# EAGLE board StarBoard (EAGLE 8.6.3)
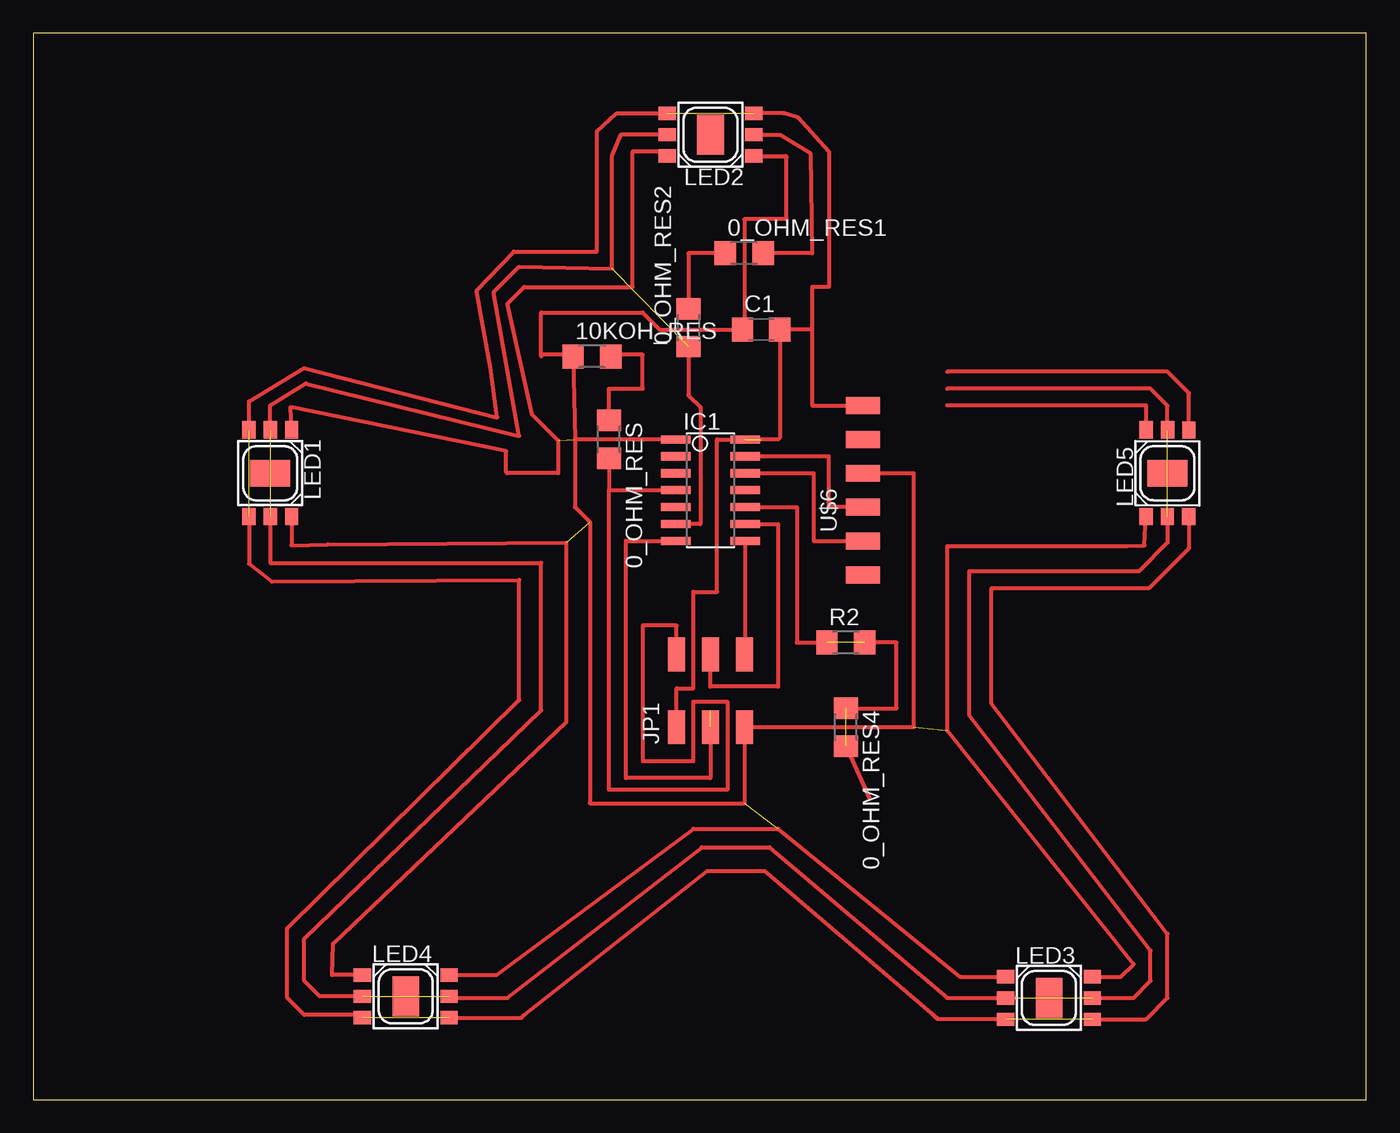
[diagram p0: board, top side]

Size 100 x 80 mm. Coordinates in mm from the lower left corner, seen from the top.
Outline: 0,0 100,0 100,80 0,80 0,0
Copper layers (1*16): Top 0.035mm / dielectric 1.5mm / Bottom 0.035mm
Design rules "default": minimum track width 6mil, minimum drill 0.35mm, track to track 6mil, track to pad 6mil, pad to pad 6mil, via to via 6mil, smd to smd 6mil, copper to edge 40mil, drill to drill 6mil, minimum pad ring 10mil, minimum via ring 8mil, stop-mask expansion 4mil, vias tented up to drill 0mil, thermal gap 10mil

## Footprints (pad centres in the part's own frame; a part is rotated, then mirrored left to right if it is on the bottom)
R1206 = smd 1.6 x 1.803: 1 -1.422,0; 2 1.422,0
C1206 = smd 1.6 x 1.8: 1 -1.4,0; 2 1.4,0
SOIC14 = smd 0.61 x 2.21: 1 -3.81,-2.603; 2 -2.54,-2.603; 3 -1.27,-2.603; 4 0,-2.603; 5 1.27,-2.603; 6 2.54,-2.603; 7 3.81,-2.603; 8 3.81,2.603; 9 2.54,2.603; 10 1.27,2.603; 11 0,2.603; 12 -1.27,2.603; 13 -2.54,2.603; 14 -3.81,2.603
2X03SMD = smd 2.54 x 1.27: 1 -2.54,2.54; 2 2.92,2.54; 3 -2.54,0; 4 2.92,0; 5 -2.54,-2.54; 6 2.92,-2.54
LP2C63-ST-RGB-SR0 = smd 1.3 x 1: 1 -3.25,1.6; 2 -3.25,0; 3 -3.25,-1.6; 4 3.25,-1.6; 5 3.25,0; 6 3.25,1.6 | smd 2 x 3: TH 0,0
1X06SMD = smd 2.54 x 1.27: 1 0,6.35; 2 0,3.81; 3 0,1.27; 4 0,-1.27; 5 0,-3.81; 6 0,-6.35

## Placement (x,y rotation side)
0_OHM_RES  [R1206]  43.18,49.53 270 top
0_OHM_RES1  [R1206]  53.34,63.5 0 top
0_OHM_RES2  [R1206]  49.15,57.91 90 top
0_OHM_RES4  [R1206]  60.96,27.94 270 top
10KOH_RES  [R1206]  41.91,55.75 0 top
C1  CAP-US1206  [C1206]  54.61,57.78 0 top
IC1  ATTINY44-SSU  [SOIC14]  50.8,45.72 270 top
JP1  [2X03SMD]  50.8,30.48 90 top
LED1  LP2C63-ST-RGB-SR0  [LP2C63-ST-RGB-SR0]  17.78,46.99 270 top
LED2  LP2C63-ST-RGB-SR0  [LP2C63-ST-RGB-SR0]  50.8,72.39 180 top
LED3  LP2C63-ST-RGB-SR0  [LP2C63-ST-RGB-SR0]  76.2,7.62 0 top
LED4  LP2C63-ST-RGB-SR0  [LP2C63-ST-RGB-SR0]  27.94,7.75 0 top
LED5  LP2C63-ST-RGB-SR0  [LP2C63-ST-RGB-SR0]  85.09,46.99 89.9 top
R2  [R1206]  60.96,34.29 0 top
U$6  FTDI-SMD-HEADER  [1X06SMD]  62.23,45.72 0 top

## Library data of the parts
0_OHM_RES 0_OHM_RES1 0_OHM_RES2 0_OHM_RES4 10KOH_RES C1 IC1 JP1 R2 U$6 = fab
LED1-LED5 = led

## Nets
GND: C1.2 IC1.14 JP1.1 LED1.3 LED1.4 LED2.3 LED2.4 LED3.3 LED3.4 LED4.3 LED4.4 LED5.3 U$6.1
N$1: IC1.8 JP1.6
N$5: 0_OHM_RES.1 10KOH_RES.2
N$7: IC1.12 U$6.5
N$8: IC1.13 U$6.4
N$9: IC1.7 JP1.3
N$10: IC1.9 JP1.4
N$16: LED5.6
N$19: 0_OHM_RES1.2 LED2.2
N$24: 0_OHM_RES1.1 0_OHM_RES2.2
N$26: LED5.4
PA3: 0_OHM_RES4.1 0_OHM_RES4.2 IC1.10 R2.1 R2.2
PA7: 0_OHM_RES2.1 IC1.6 LED1.2 LED1.5 LED2.5 LED3.2 LED3.5 LED4.2 LED4.5 LED5.2 LED5.5
REST: 0_OHM_RES.2 IC1.4 JP1.2
VCC: 10KOH_RES.1 C1.1 IC1.1 JP1.5 LED1.1 LED1.6 LED2.1 LED2.6 LED3.1 LED3.6 LED4.1 LED4.6 LED5.1 U$6.3

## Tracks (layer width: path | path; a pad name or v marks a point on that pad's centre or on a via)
GND  (5 unrouted)
  Top 0.305: IC1.14 51.31,49.53 51.31,38.1 49.53,38.1 49.53,30.86 48.26,30.86 JP1.1 | 54.61,49.53 55.88,49.53 56.01,49.66 C1.2 58.42,57.78 | 58.42,57.78 58.42,60.96 59.69,60.96 59.69,71.12 57.4,73.66 56.31,73.99 LED2.3 | 58.42,57.78 58.42,52.07 U$6.1 | LED1.3 16.18,52.38 20.32,54.86 34.8,51.18 34.29,54.86 33.27,60.71 36.07,63.63 42.29,63.63 42.29,72.64 43.76,73.99 LED2.4 | LED4.3 24.49,6.35 20.32,6.35 19.05,7.62 19.05,12.83 36.45,29.97 36.45,38.99 17.91,38.86 16.18,40.21 LED1.4 | LED4.4 36.63,6.15 36.83,6.35 50.55,17.14 54.86,17.14 67.4,6.45 | 67.82,6.1 67.4,6.45 | LED3.3 67.83,6.02 67.4,6.45 | LED3.4 83.49,6.02 85.09,7.62 85.09,12.45 71.88,29.72 71.88,38.35 83.69,38.35 86.68,41.34 LED5.3 86.36,43.41
N$1
  Top 0.305: IC1.8 53.4,33.4 JP1.6
N$5
  Top 0.305: 0_OHM_RES.1 43.18,53.34 45.72,53.34 45.72,55.88 43.46,55.88 10KOH_RES.2
N$7
  Top 0.305: IC1.12 58.55,46.99 58.55,41.91 U$6.5
N$8
  Top 0.305: U$6.4 59.69,44.45 59.69,48.26 IC1.13
N$9  (1 unrouted)
  Top 0.305: JP1.3 50.8,24.13 44.45,24.13 44.45,41.91 IC1.7
N$10
  Top 0.305: IC1.9 55.88,43.18 55.88,30.99 50.8,30.99 JP1.4
N$16
  Top 0.305: LED5.6 83.5,52.07 68.58,52.07
N$19
  Top 0.305: LED2.2 56.01,72.39 58.29,70.99 58.42,63.5 0_OHM_RES1.2
N$24
  Top 0.305: 0_OHM_RES1.1 49.15,63.5 0_OHM_RES2.2
N$26
  Top 0.305: LED5.4 86.7,53 85.09,54.61 68.58,54.61
PA3  (2 unrouted)
  Top 0.305: IC1.10 57.28,44.45 57.28,34.29 R2.1 | R2.2 64.77,34.29 64.77,29.36 0_OHM_RES4.1 | 0_OHM_RES4.2 62.74,22.61
PA7  (5 unrouted)
  Top 0.305: IC1.6 50.04,43.18 50.04,51.94 49.15,52.83 0_OHM_RES2.1 | LED2.5 44.07,72.39 43.43,70.87 43.43,62.36 36.45,62.48 34.54,60.58 36.45,49.78 20.45,53.72 17.78,52.07 LED1.2 | LED4.2 21.46,7.75 20.32,8.89 20.32,12.06 38.1,29.21 38.1,40.26 17.78,40.26 LED1.5 | LED4.5 31.32,7.62 35.56,7.62 50.16,18.92 55.24,18.92 68.58,7.62 LED3.2 73.66,7.62 | LED3.5 82.55,7.62 83.82,8.89 83.82,11.18 70.23,28.83 70.23,39.62 82.93,39.62 85.08,41.78 LED5.2 | LED5.5 85.1,52.06 83.82,53.34 68.58,53.34
REST
  Top 0.305: 0_OHM_RES.2 43.18,45.72 | 43.18,45.72 IC1.4 | JP1.2 48.26,35.56 45.72,35.56 45.72,25.4 49.53,25.4 49.53,29.84 52.07,29.84 52.07,23.24 43.18,23.24 43.18,45.72
VCC  (4 unrouted)
  Top 0.305: U$6.3 66.04,46.99 66.04,27.94 JP1.5 53.34,22.23 41.76,22.23 41.76,43.33 40.64,44.45 40.64,49.53 | 38.1,55.75 38.1,55.88 | 38.1,55.88 38.1,59.05 45.72,59.05 46.99,57.78 C1.1 53.34,57.78 53.34,66.04 56.52,66.04 56.52,70.74 56.46,70.79 LED2.1 | 40.64,49.53 10KOH_RES.1 40.36,55.88 38.1,55.88 | IC1.1 40.64,49.53 | LED2.6 47.22,71.12 44.96,71.12 44.96,60.96 36.83,60.96 35.56,59.69 37.4,51.41 39.37,49.44 39.37,46.99 35.56,46.99 35.48,47.07 35.48,48.65 19.3,51.94 LED1.1 | LED4.1 22.4,9.35 22.48,11.68 40.01,28.32 40.01,41.78 22.1,41.66 19.38,41.58 LED1.6 | LED4.6 34.75,9.35 49.53,20.32 55.88,20.32 69.52,9.22 LED3.1 | LED3.6 81.61,9.22 82.55,10.16 68.58,27.69 68.58,41.53 82.04,41.53 83.36,41.57 LED5.1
